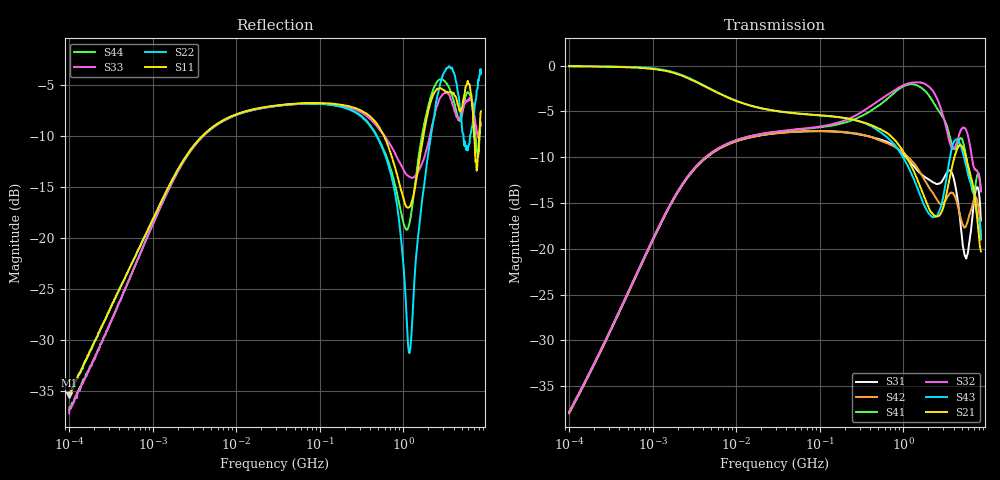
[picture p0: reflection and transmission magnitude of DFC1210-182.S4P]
# Hz S dB R 50
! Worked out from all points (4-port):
!   801 points, 100 kHz to 8.5 GHz, reference 50 ohm
!   strongest paths, dB at 100 kHz, 1.721 MHz, 29.51 MHz, 502.3 MHz, 8.5 GHz:
!     S21: -0.1, -0.8, -4.9, -6.8, -20.3
!     S43: -0.1, -0.7, -5.0, -7.1, -18.8
!     S32: -37.8, -14.7, -7.2, -3.8, -13.7
!     S41: -37.9, -14.7, -7.2, -4.4, -13.7
!     S42: -38.0, -14.8, -7.4, -8.1, -19.0
!     S31: -37.9, -14.8, -7.4, -8.0, -16.9
!   lowest |S11| = -35.5 dB at 100 kHz (marker M1), VSWR 1.03, Z = 50.5 + j1.62 ohm
!   |S11| at or under -10 dB: start of sweep to 3.94 MHz; 587.8 MHz to 1.742 GHz (1.154 GHz wide, 99.1 % of centre); 7.042 GHz to 8.1 GHz (1.058 GHz wide, 14 % of centre)
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100000  -35.48 72.1  -0.07 -0.9  -37.92 -99.3  -37.85 80.5
        -0.07 -0.9  -35.37 72.4  -37.88 80.9  -37.92 -99.6
        -37.88 -99.8  -37.84 80.5  -37.23 71.6  -0.09 -0.8
        -37.85 80.6  -37.96 -100.0  -0.09 -0.8  -36.93 75.3
7878354  -8.24 24.3  -3.48 -14.7  -8.61 -155.2  -8.50 26.2
         -3.48 -14.7  -8.26 24.2  -8.50 26.3  -8.62 -155.2
         -8.62 -155.2  -8.52 26.3  -8.31 25.0  -3.44 -14.9
         -8.52 26.2  -8.63 -155.2  -3.44 -15.0  -8.31 25.1
3.903248e8  -8.00 -17.0  -6.41 -33.6  -7.73 142.9  -5.05 14.2
            -6.41 -33.7  -8.89 -16.7  -4.53 15.2  -7.72 143.1
            -7.74 142.9  -4.54 15.2  -8.26 -18.7  -6.50 -35.8
            -5.06 14.2  -7.73 143.1  -6.50 -35.8  -8.82 -18.5
1.187242e9  -16.99 9.7  -10.58 -89.1  -10.44 82.9  -2.05 -1.2
            -10.59 -89.1  -31.33 33.1  -1.91 -0.2  -10.14 84.3
            -10.45 82.9  -1.92 -0.2  -14.01 -5.9  -11.33 -89.2
            -2.05 -1.2  -10.14 84.3  -11.33 -89.2  -18.58 27.0
2.804235e9  -5.33 55.1  -16.17 163.7  -12.79 21.4  -5.26 -27.0
            -16.17 163.7  -4.74 19.6  -4.62 -33.8  -15.09 21.0
            -12.79 21.5  -4.62 -33.7  -6.21 60.5  -15.48 172.7
            -5.26 -27.0  -15.09 21.1  -15.48 172.8  -4.44 41.6
5.01213e9  -7.29 6.1  -8.75 58.1  -18.43 -153.5  -8.00 -24.5
           -8.76 58.2  -8.87 58.0  -6.89 -16.2  -17.08 -129.3
           -18.47 -153.5  -6.89 -16.2  -7.84 1.2  -9.09 48.7
           -7.99 -24.5  -17.04 -129.1  -9.09 48.8  -8.02 4.8
8.5e9  -7.59 9.2  -20.32 -7.0  -16.91 -26.4  -13.74 -67.7
       -20.29 -7.2  -3.92 35.1  -13.69 -78.4  -19.01 -16.1
       -16.92 -26.5  -13.72 -78.4  -8.71 3.9  -18.93 -20.8
       -13.72 -67.7  -19.00 -16.3  -18.81 -20.8  -8.94 4.5
